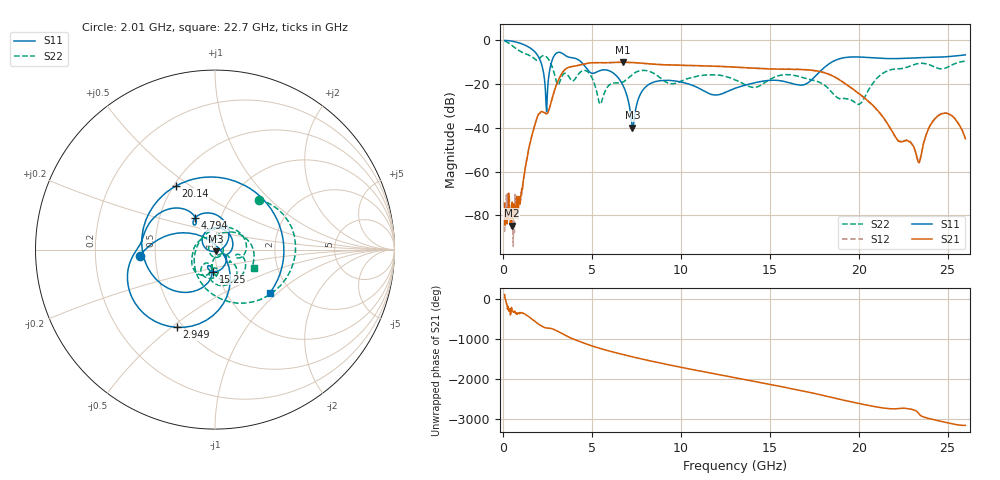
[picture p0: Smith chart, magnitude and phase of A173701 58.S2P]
!  2-Port S-parameters saved by WinCal
! VAR MeasName=S-Parameters (CALIBRATED_DATA) read from VNA (N5245A)
! VAR MeasDate=2017-6-7 10:32:16
! VAR NAME=A173701 58
! VAR FILENAME=A173701 58.S2P
! VAR DATE=2017-6-7 10:32:16
! VAR PHYS_PORTS=1,2
# Hz S DB R 50
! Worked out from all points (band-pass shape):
!   801 points, 100 MHz to 26 GHz, reference 50 ohm
!   highest |S21| = -9.97 dB at 6.769 GHz (marker M1); lowest = -84.6 dB at 488.5 MHz (marker M2)
!   |S21| within 3 dB of the highest: 3.546 GHz to 14.82 GHz (11.27 GHz wide, 123 % of centre)
!   lowest |S11| = -39.8 dB at 7.287 GHz (marker M3), VSWR 1.02, Z = 50.3 - j0.981 ohm
!   |S11| at or under -10 dB: 2.143 GHz to 2.733 GHz (590.3 MHz wide, 24.2 % of centre); 4.421 GHz to 18.47 GHz (14.05 GHz wide, 123 % of centre)
!   |S22| runs from -29.2 to -0.2 dB; largest |S21 - S12| = 0.0037
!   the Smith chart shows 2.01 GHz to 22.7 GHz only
!   S11 on the Smith chart (normalised r, x): 2.01 GHz: 0.41, -0.03; 2.949 GHz: 0.46, -0.52; 4.794 GHz: 0.76, +0.28; 15.25 GHz: 0.95, -0.24; 20.14 GHz: 0.51, +0.44; 22.7 GHz: 1.57, -0.89
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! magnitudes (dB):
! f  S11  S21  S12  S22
! 100 MHz  0.0  -74.4  -87.6  -0.2
! 488.5 MHz  -0.3  -84.6  -86.2  -2.2
! 909.4 MHz  -1.1  -71.4  -74.1  -4.6
! 2.01 GHz  -7.6  -33.7  -33.7  -8.7
! 2.463 GHz  -32.6  -33.6  -33.5  -7.6
! 2.949 GHz  -6.3  -21.8  -21.7  -16.9
! 4.438 GHz  -10.1  -11.0  -11.0  -14.0
! 4.794 GHz  -13.7  -10.4  -10.4  -14.5
! 5.474 GHz  -13.7  -10.2  -10.2  -29.2
! 6.769 GHz  -20.8  -10.0  -10.0  -19.0
! 7.287 GHz  -39.8  -10.1  -10.1  -15.6
! 7.838 GHz  -23.1  -10.5  -10.5  -13.7
! 8.744 GHz  -18.5  -11.0  -11.0  -16.5
! 13.05 GHz  -21.9  -12.2  -12.2  -18.0
! 15.25 GHz  -18.2  -13.1  -13.0  -16.9
! 17.39 GHz  -17.8  -13.7  -13.6  -18.1
! 20.14 GHz  -7.6  -25.0  -25.2  -28.5
! 21.69 GHz  -8.3  -39.1  -39.0  -13.7
! 22.7 GHz  -8.2  -45.7  -45.5  -12.3
! 23.41 GHz  -7.9  -55.9  -55.2  -10.5
! 24.8 GHz  -7.5  -33.3  -33.1  -12.9
! 26 GHz  -6.6  -44.9  -44.8  -9.5
